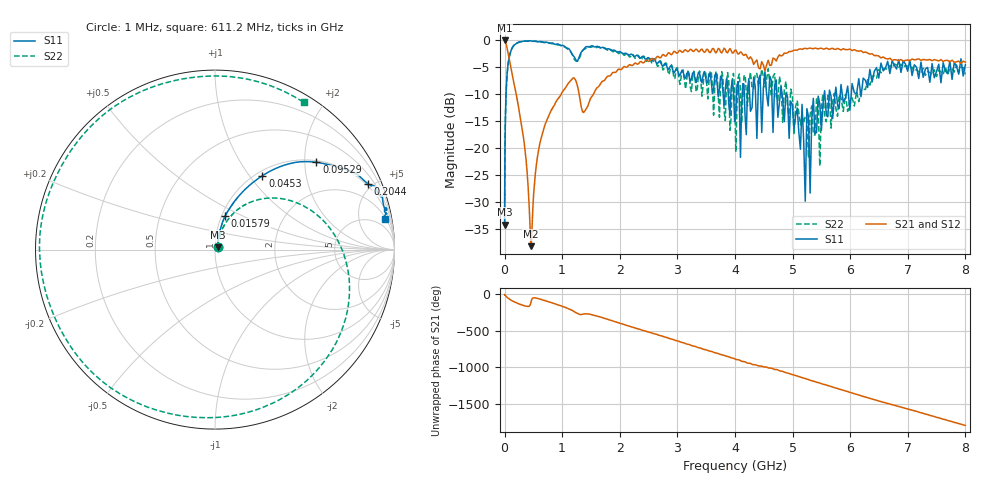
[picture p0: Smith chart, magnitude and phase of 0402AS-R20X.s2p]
!s-Parameter Generated by FASTRON Sdn. Bhd.
!FASTRON P/N : 0402AS-R20X
!Keysight Technologies: E5071C_MY46733604_B.14.02
!Date: Mon Dec 01 10:50:03 2025
!Version  :Rev00  Mon Dec 01 10:50:03 2025
!Data & Calibration Information:
!Freq  S11:SOLT2(ON)  S21:SOLT2(ON)  S12:SOLT2(ON)  S22:SOLT2(ON)
!PortZ  Port1:50+j0  Port2:50+j0
!When reading reference impedance value at option line is always used.
! Remarks : This data is being provided solely for informational purposes.
# Hz S dB R 50
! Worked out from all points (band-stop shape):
!   1601 points, 1 MHz to 8 GHz, reference 50 ohm
!   highest |S21| = -0.10 dB at 6.268 MHz (marker M1); lowest = -38.1 dB at 457.7 MHz (marker M2)
!   |S21| within 3 dB of the highest: 2.722 GHz to 4.212 GHz (1.49 GHz wide, 43 % of centre); 4.751 GHz to 6.51 GHz (1.759 GHz wide, 31.2 % of centre)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
!   lowest |S11| = -34.1 dB at 1.013 MHz (marker M3), VSWR 1.04, Z = 51.5 + j1.36 ohm
!   |S11| at or under -10 dB: 4.068 GHz to 4.127 GHz (58.54 MHz wide, 1.43 % of centre); 4.892 GHz to 5.549 GHz (656.6 MHz wide, 12.6 % of centre); 5.658 GHz to 5.737 GHz (78.88 MHz wide, 1.38 % of centre)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
!   |S22| runs from -34.2 to -0.2 dB; largest |S21 - S12| = 0.015
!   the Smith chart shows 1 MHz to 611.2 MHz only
!   S11 on the Smith chart (normalised r, x): 1 MHz: 1.03, +0.03; 15.79 MHz: 1.04, +0.41; 45.3 MHz: 1.07, +1.16; 95.29 MHz: 1.04, +2.29; 204.4 MHz: 0.90, +4.66; 611.2 MHz: 2, +11
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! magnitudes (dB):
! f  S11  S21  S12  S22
! 1 MHz  -33.9  -0.1  -0.1  -33.8
! 1.013 MHz  -34.1  -0.1  -0.1  -33.9
! 4.479 MHz  -24.5  -0.2  -0.1  -24.5
! 6.268 MHz  -21.8  -0.1  -0.1  -21.9
! 15.79 MHz  -14.1  -0.4  -0.4  -14.1
! 20.07 MHz  -12.1  -0.5  -0.5  -12.1
! 45.3 MHz  -6.2  -1.6  -1.6  -6.3
! 89.95 MHz  -2.8  -4.0  -4.0  -2.8
! 95.29 MHz  -2.6  -4.3  -4.3  -2.5
! 204.4 MHz  -0.7  -10.2  -10.2  -0.7
! 312.6 MHz  -0.3  -16.9  -16.9  -0.3
! 400.7 MHz  -0.2  -25.7  -25.7  -0.2
! 457.7 MHz  -0.2  -38.1  -38.1  -0.2
! 611.2 MHz  -0.3  -19.2  -19.2  -0.4
! 1.154 GHz  -2.3  -7.5  -7.5  -2.3
! 1.388 GHz  -1.5  -13.2  -13.2  -1.7
! 1.795 GHz  -1.6  -6.7  -6.7  -1.9
! 3.974 GHz  -9.2  -2.4  -2.4  -6.2
! 4.577 GHz  -12.2  -3.8  -3.8  -5.3
! 5.164 GHz  -11.9  -1.8  -1.8  -14.1
! 6.651 GHz  -4.0  -3.5  -3.5  -5.5
! 8 GHz  -4.6  -4.1  -4.1  -6.4
